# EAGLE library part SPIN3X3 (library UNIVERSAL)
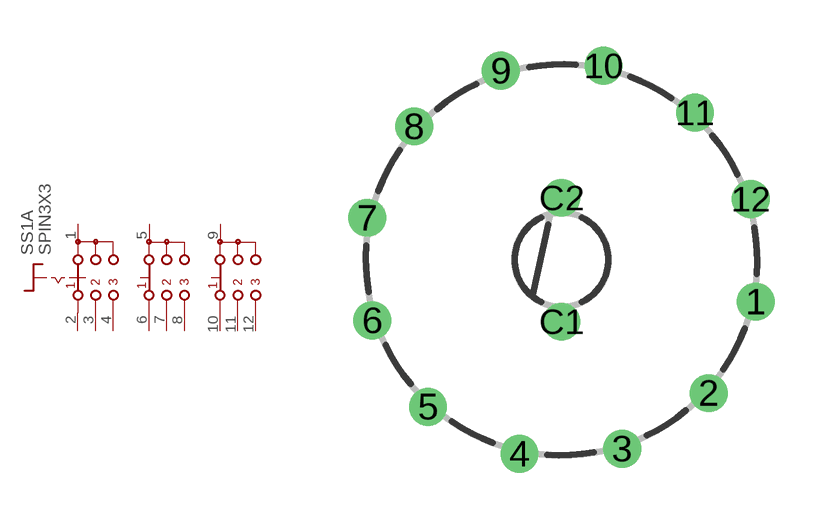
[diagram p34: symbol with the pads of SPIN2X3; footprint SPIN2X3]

Designator prefix S; gates S1A=SPIN2X3 S1B=SPIN2X3B S1C=SPIN2X3B

## SPIN3X3  [SPIN2X3]
1  S1A:A  pas
2  S1A:A1  pas
3  S1A:A2  pas
4  S1A:A3  pas
5  S1B:B  pas
6  S1B:B1  pas
7  S1B:B2  pas
8  S1B:B3  pas
9  S1C:B  pas
10  S1C:B1  pas
11  S1C:B2  pas
12  S1C:B3  pas

## Footprint SPIN2X3 (pad centres in mm)
drill 0.7 pad 1.2: 1 6.207,-1.342; 2 4.704,-4.265; 3 1.941,-6.046; 4 -1.342,-6.207; 5 -4.265,-4.704; 6 -6.046,-1.941; 7 -6.207,1.342; 8 -4.704,4.265; 9 -1.941,6.046; 10 1.342,6.207; 11 4.265,4.704; 12 6.046,1.941; C1 0,-1.98; C2 0,1.98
